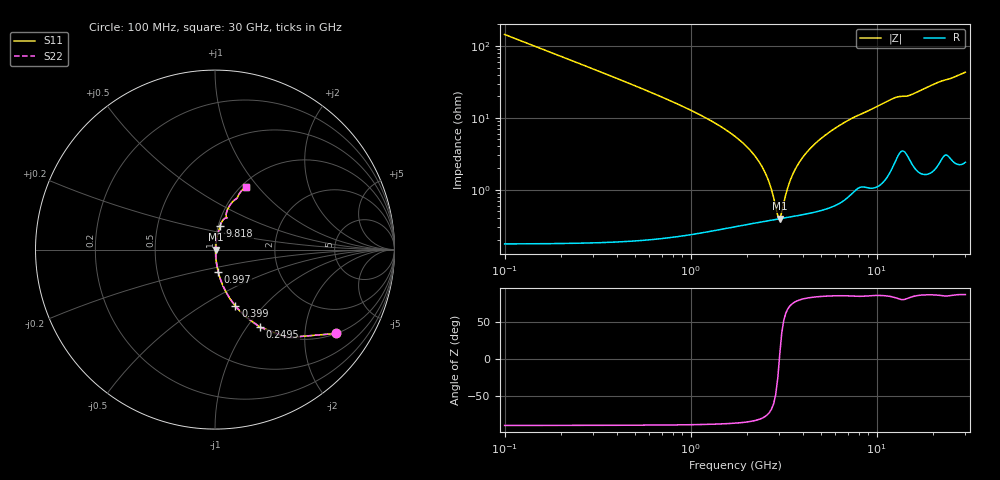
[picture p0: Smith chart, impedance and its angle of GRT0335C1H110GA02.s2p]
!Murata Part Number: GRT0335C1H110GA02
!These Parameters are Measured in Series Mode Connection
!Data Generated on Jun 19, 2026
!  o--ll--o
!Port1  Port2
!  o------o
!Operation Temp=25[degC], DC Bias Voltage=0[V]
!Freq. Start=100[MHz] Stop=30[GHz] 401[Steps]
# Hz S RI R 50
!Freq.(Hz) S11(Real) S11(Imag) S21(Real) S21(Imag) S12(Real) S12(Imag) S22(Real) S22(Imag)
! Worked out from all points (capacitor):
!   401 points, 100 MHz to 30 GHz, reference 50 ohm
!   read as one part in series: C = 11 pF near 249.5 MHz
!   lowest |Z| = 397 mohm at 3.015 GHz (marker M1)
!   series resonance near 3.001 GHz, so ESL is about 260 pH
!   S11 on the Smith chart (normalised r, x): 100 MHz: 1.00, -2.89; 249.5 MHz: 1.00, -1.15; 399 MHz: 1.00, -0.71; 997 MHz: 1.00, -0.26; 9.818 GHz: 1.02, +0.28; 30 GHz: 1.05, +0.86
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1e8  0.676 -0.4674  0.324 0.4674  0.324 0.4674  0.676 -0.4674
2.495e8  0.2496 -0.4312  0.7504 0.4312  0.7504 0.4312  0.2496 -0.4312
3.99e8  0.1137 -0.3148  0.8863 0.3148  0.8863 0.3148  0.1137 -0.3148
6.2325e8  0.0486 -0.2104  0.9514 0.2104  0.9514 0.2104  0.0486 -0.2104
9.97e8  0.0185 -0.1258  0.9815 0.1258  0.9815 0.1258  0.0185 -0.1258
2.26775e9  0.00418 -0.0268  0.9958 0.0268  0.9958 0.0268  0.00418 -0.0268
2.56675e9  0.00388 -0.0148  0.9961 0.0148  0.9961 0.0148  0.00388 -0.0148
2.86575e9  0.00386 -0.00433  0.9961 0.00433  0.9961 0.00433  0.00386 -0.00433
3.01525e9  0.00393 0.000467  0.9961 -0.000467  0.9961 -0.000467  0.00393 0.000467
3.09e9  0.00398 0.00278  0.996 -0.00278  0.996 -0.00278  0.00398 0.00278
3.46375e9  0.00436 0.0136  0.9956 -0.0136  0.9956 -0.0136  0.00436 0.0136
3.76275e9  0.0048 0.0215  0.9952 -0.0215  0.9952 -0.0215  0.0048 0.0215
4.286e9  0.00581 0.0343  0.9942 -0.0343  0.9942 -0.0343  0.00581 0.0343
5.10825e9  0.00794 0.0525  0.9921 -0.0525  0.9921 -0.0525  0.00794 0.0525
7.05175e9  0.0161 0.0902  0.9839 -0.0902  0.9839 -0.0902  0.0161 0.0902
9.8175e9  0.029 0.134  0.971 -0.134  0.971 -0.134  0.029 0.134
1.01165e10  0.0309 0.1391  0.9691 -0.1391  0.9691 -0.1391  0.0309 0.1391
1.25085e10  0.0552 0.174  0.9448 -0.174  0.9448 -0.174  0.0552 0.174
1.505e10  0.0624 0.1865  0.9376 -0.1865  0.9376 -0.1865  0.0624 0.1865
2.005825e10  0.091 0.2582  0.909 -0.2582  0.909 -0.2582  0.091 0.2582
2.50665e10  0.129 0.2997  0.871 -0.2997  0.871 -0.2997  0.129 0.2997
3e10  0.1702 0.3488  0.8298 -0.3488  0.8298 -0.3488  0.1702 0.3488
